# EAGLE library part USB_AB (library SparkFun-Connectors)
USB Type AB Micro Connector OTG-compatible. 5 pins, 3 shield pins SparkFun Products: IOIO-OTG SparkFun SAMD21 Mini Breakout
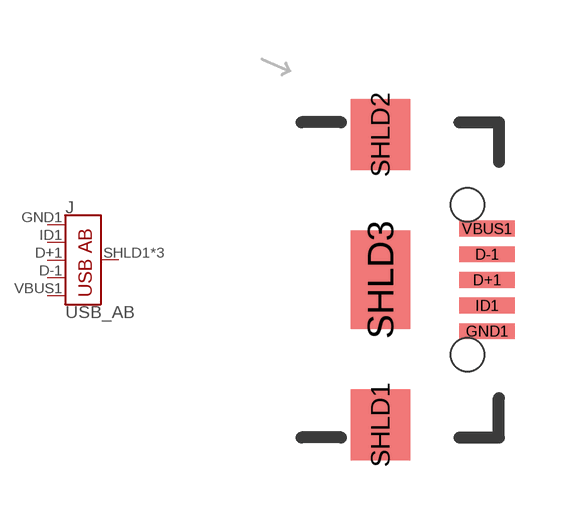
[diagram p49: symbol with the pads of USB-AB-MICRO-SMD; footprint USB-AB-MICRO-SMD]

Designator prefix J

## USB_AB_SMT (PROD_ID: CONN-11794)  [USB-AB-MICRO-SMD]
D+1  D+
D-1  D-
GND1  GND  pwr
ID1  USBID
SHLD1  SHIELD
SHLD2  SHIELD
SHLD3  SHIELD
VBUS1  VBUS  pwr

## Footprint USB-AB-MICRO-SMD (pad centres in mm)
USB Type AB - SMT Basic silk outline Specifications: Pin count:5 main, 3 shield Datasheet referenced for footprint: http://www.morethanall.com//upload/products_pdf/87340574052ba5151280ca.pdf Example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
smd 1.4 x 0.4: D+1 2.7,0; D-1 2.7,0.65; GND1 2.7,-1.3; ID1 2.7,-0.65; VBUS1 2.7,1.3
smd 1.5 x 1.8: SHLD1 0,-3.68; SHLD2 0,3.68
smd 1.5 x 2.5: SHLD3 0,0
hole 0.85 at 2.2,1.9
hole 0.85 at 2.2,-1.9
